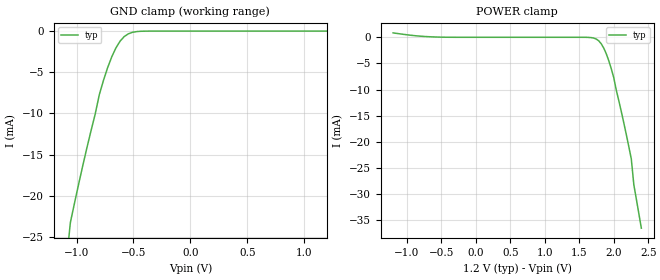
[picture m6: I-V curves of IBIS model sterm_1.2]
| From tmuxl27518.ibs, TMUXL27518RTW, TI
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| sterm_1.2
[Model]   sterm_1.2
Model_type   Terminator
|   typ   min   max
C_comp   1.598234e-12   NA   NA
[Voltage Range]   1.2   NA   NA
[Temperature Range]   27   NA   NA
[Power Clamp Reference]   1.2   NA   NA
[GND Clamp Reference]   0   NA   NA
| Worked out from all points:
|   GND clamp passes 1 mA (typ) near -0.60 V on its own axis
[GND Clamp]
|   Voltage   I(typ)   I(min)   I(max)
-2.4V     -146.9mA   NA         NA
-1.091V   -28.16mA   NA         NA
-1.055V   -23.26mA   NA         NA
-909.1mV  -14.17mA   NA         NA
-800mV    -7.715mA   NA         NA
-763.6mV  -5.992mA   NA         NA
-690.9mV  -3.133mA   NA         NA
-654.5mV  -2.054mA   NA         NA
-618.2mV  -1.236mA   NA         NA
-545.5mV  -333.4uA   NA         NA
-400mV    -8.925uA   NA         NA
1.2V      184.3pA    NA         NA
[POWER Clamp]
|   Voltage   I(typ)   I(min)   I(max)
-1.2V     837.9uA    NA         NA
-509.1mV  26.66uA    NA         NA
1.636V    -24.62uA   NA         NA
1.782V    -674.3uA   NA         NA
1.855V    -2.054mA   NA         NA
1.891V    -3.133mA   NA         NA
2V        -7.715mA   NA         NA
2.036V    -10.09mA   NA         NA
2.145V    -16.34mA   NA         NA
2.255V    -23.26mA   NA         NA
2.291V    -28.16mA   NA         NA
2.4V      -36.49mA   NA         NA
